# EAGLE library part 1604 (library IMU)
Adafruit 10-DOF IMU Breakout - L3GD20H + LSM303 + BMP180
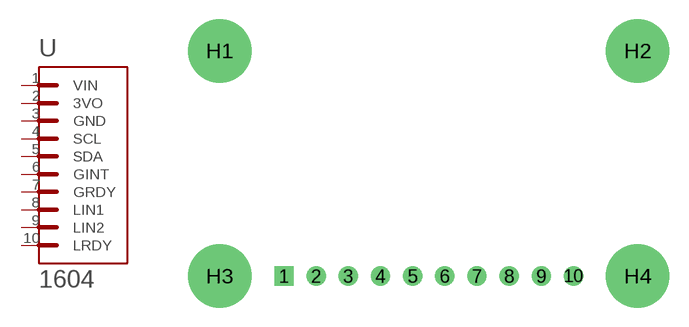
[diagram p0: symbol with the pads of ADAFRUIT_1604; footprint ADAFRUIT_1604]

Designator prefix -

## 1604 (Availability: Bad; Description: Adafruit 10-DOF IMU Breakout - L3GD20H + LSM303 + BMP180; MF: Adafruit Industries; MP: 1604; Package: None; Price: 26.66 USD)  [ADAFRUIT_1604]
1  VIN  pwr
2  3VO  pwr
3  GND  pwr
4  SCL
5  SDA
6  GINT  out
7  GRDY  out
8  LIN1  out
9  LIN2  out
10  LRDY  out

## Footprint ADAFRUIT_1604 (pad centres in mm)
drill 1.016 square: 1 -11.43,-0.001
drill 1.016: 2 -8.89,-0.001; 3 -6.35,-0.001; 4 -3.81,-0.001; 5 -1.27,-0.001; 6 1.27,-0.001; 7 3.81,-0.001; 8 6.35,-0.001; 9 8.89,-0.001; 10 11.43,-0.001
drill 4: H1 -16.512,17.779; H2 16.509,17.778; H3 -16.511,0; H4 16.509,0

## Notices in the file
This work is licensed under a Creative Commons Attribution-ShareAlike 4.0 International License (CC BY-SA) with Design Exception 1.0
